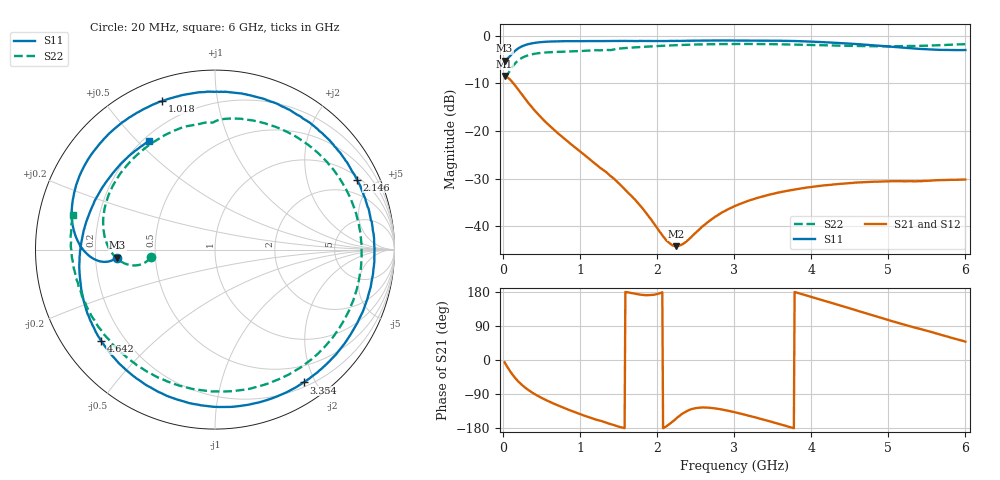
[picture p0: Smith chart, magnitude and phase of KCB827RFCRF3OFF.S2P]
!Agilent Technologies,E5071B,JP1KK00126,A.08.11
!Date: Tue May 06 07:24:10 2014
!Data & Calibration Information:
!Freq	S11:SOLT2(ON)	S21:SOLT2(ON)	S12:SOLT2(ON)	S22:SOLT2(ON)
# Hz S dB R 50
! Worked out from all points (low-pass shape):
!   600 points, 20 MHz to 6 GHz, reference 50 ohm
!   highest |S21| = -8.44 dB at 20 MHz (marker M1); lowest = -44.2 dB at 2.246 GHz (marker M2)
!   |S21| within 3 dB of the highest: start of sweep to 203.2 MHz
!   lowest |S11| = -5.2 dB at 20 MHz (marker M3), VSWR 3.41, Z = 14.7 - j1.84 ohm
!   |S11| at or under -10 dB: nowhere
!   |S22| runs from -8.9 to -1.7 dB; largest |S21 - S12| = 0.00095
!   S11 on the Smith chart (normalised r, x): 20 MHz: 0.29, -0.04; 1.018 GHz: 0.10, +0.70; 2.146 GHz: 1.13, +3.98; 3.354 GHz: 0.26, -1.84; 4.642 GHz: 0.12, -0.35; 6 GHz: 0.22, +0.54
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2e7  -5.24 -175.4  -8.44 -6.0  -8.43 -6.0  -8.90 -173.1
1.697496e8  -2.97 -177.8  -10.72 -50.5  -10.71 -50.4  -5.56 -172.7
2.795659e8  -1.99 172.0  -13.11 -71.7  -13.09 -71.7  -4.37 176.6
4.093489e8  -1.50 159.7  -15.68 -89.8  -15.66 -89.8  -3.78 164.1
7.088481e8  -1.17 134.1  -20.43 -119.6  -20.42 -119.6  -3.38 139.6
1.018331e9  -1.13 109.6  -24.53 -144.2  -24.53 -144.3  -3.20 117.0
1.237963e9  -1.10 92.9  -27.45 -159.1  -27.45 -159.0  -3.04 101.2
1.497529e9  -1.10 73.6  -30.91 -175.6  -30.90 -175.5  -2.70 84.6
1.747112e9  -1.10 55.3  -35.05 173.6  -35.01 173.6  -2.41 66.8
2.016661e9  -1.10 35.7  -40.77 174.9  -40.75 175.0  -2.14 48.2
2.146444e9  -1.09 26.3  -43.37 -171.0  -43.37 -171.1  -2.04 39.5
2.246277e9  -1.08 19.2  -44.18 -154.8  -44.16 -154.6  -1.97 33.1
2.615659e9  -1.01 -6.6  -39.69 -125.4  -39.70 -125.6  -1.79 9.7
3.014992e9  -1.00 -33.9  -35.72 -138.4  -35.71 -138.3  -1.72 -14.5
3.354424e9  -1.02 -56.3  -33.80 -155.9  -33.81 -156.0  -1.74 -34.2
3.693856e9  -1.07 -78.3  -32.56 -175.4  -32.54 -175.3  -1.81 -54.0
4.013322e9  -1.24 -99.0  -31.73 165.7  -31.70 165.8  -1.94 -73.3
4.312821e9  -1.48 -118.9  -31.18 147.6  -31.20 147.5  -2.05 -91.8
4.64227e9  -1.79 -141.1  -30.78 127.3  -30.78 127.4  -2.16 -112.8
5.011653e9  -2.27 -167.2  -30.57 104.8  -30.55 104.9  -2.19 -136.5
5.460902e9  -2.81 159.8  -30.48 79.3  -30.49 79.4  -2.09 -164.0
6e9  -2.99 121.5  -30.18 48.5  -30.17 48.8  -1.76 166.2
